| TEXAS INSTRUMENTS INCORPORATED
| Standard Linear and Logic Group
| IBIS Model of TS5A23157
| Dual 10 Ohm SPDT Analog Switch
| This file contains package information for the following:
|  VSSOP 10-pin (DGS) package as [Component] TS5A23157_DGS
| This device can be powered at the following Vccs:
|  5 volt Vcc
|  3.3 volt Vcc
|  2.5 volt Vcc
|  1.8 volt Vcc
| This file provides unique models under the [Model Selector] for each Vcc.
| For operation at a specific Vcc, select the appropriate model after each
| [Model Selector] keyword.
[IBIS Ver]   3.2
[Comment char]  |_char
[File Name]   ts5a23157.ibs
[File Rev]   1.1 | x_die
[Date]   September 27, 2005
[Source]   Data created from TI-SPICE simulations at TI-SLL.
[Notes]   The following is an IBIS list for the TS5A23157.
   Please contact sllibis@ti.com with questions and
   comments concerning SLL IBIS models.
   - FILE REV HISTORY
   - 1.1 Release IBIS file on 10/06/05
   - Power clamp data deleted in the IN models as there
   is no power-clamp diode.
   - Non-monotonic data due to FET characteristics.
   - NCH & PCH MOSFETS, so [Series Mosfet] model can have rising
   or falling currents
[Disclaimer] Property of Texas Instruments Incorporated.  Unauthorized
   reproduction and/or distribution is strictly prohibited.
   This product is protected under copyright law.
   Created  2005, (C) Copyright  2005, Texas Instruments
   Incorporated, All Rights Reserved
   UNLESS THERE IS A SIGNED, WRITTEN AGREEMENT TO THE
   CONTRARY, TEXAS INSTRUMENTS (TI) IS PROVIDING THE IBIS
   MODELS  AND WITHOUT ANY WARRANTY, EXPRESSED OR
   IMPLIED.  TI assumes no liability for:
   1) the accuracy of the IBIS models provided to your
   company;
   2) the proper functioning of these IBIS Models in your
   design or for any resulting applications; or
   3) infringement of patents, copyrights or intellectual
   property rights resulting from your use of these IBIS
   models.
   TI provides IBIS Models as a service to our customers.
   You and your company shall not distribute, sell or give
   these models to anyone else without prior written
   permission from TI.
   TI reserves the right to make changes to our products or
   to discontinue any semiconductor product or service
   without notice, and advises our customers to obtain the
   latest version of relevant information to verify, before
   placing orders, that the information being relied on is
   current.
   Please be aware that your receipt and use of the IBIS
   information provided shall serve as acceptance of these
   terms and conditions.  If you do not accept these terms,
   you should return or destroy the IBIS models and any
   other accompanying information immediately.
| Component TS5A23157_DGS 10-pin VSSOP
[Component]   TS5A23157_DGS
[Manufacturer]   Texas Instruments, Inc.
[Package]
|   typ   min   max
R_pkg   4.300e-02   4.100e-02   4.700e-02
L_pkg   2.235e-09   2.157e-09   2.339e-09
C_pkg   3.350e-13   3.080e-13   3.550e-13
[Pin]   signal_name   model_name   R_pin   L_pin   C_pin
1   IN1   TS5A23157_IN   4.700e-02   2.339e-09   3.100e-13
2   NO1   TS5A23157_NX   4.300e-02   2.213e-09   3.550e-13
3   GND   GND   4.100e-02   2.157e-09   3.540e-13
4   NO2   TS5A23157_NX   4.300e-02   2.213e-09   3.550e-13
5   IN2   TS5A23157_IN   4.700e-02   2.339e-09   3.100e-13
6   COM2   TS5A23157_COM   4.500e-02   2.284e-09   3.080e-13
7   NC2   TS5A23157_NX   4.100e-02   2.176e-09   3.500e-13
8   VCC   POWER   4.100e-02   2.172e-09   3.500e-13
9   NC1   TS5A23157_NX   4.100e-02   2.176e-09   3.510e-13
10   COM1   TS5A23157_COM   4.500e-02   2.284e-09   3.080e-13
[Series Switch Groups]
| Function Group States
On  1 /   | NC1->COM1 IN1 LOW
On  2 /   | NO1->COM1 IN1 HIGH
On  3 /   | NC2->COM2 IN2 LOW
On  4 /   | NO2->COM2 IN2 HIGH
On  5 /   | COM1->NC1 IN1 LOW
On  6 /   | COM1->NO1 IN1 HIGH
On  7 /   | COM2->NC2 IN2 LOW
On  8 /   | COM2->NO2 IN2 HIGH
Off 1 /   | IN1 HIGH
Off 2 /   | IN1 LOW
Off 3 /   | IN2 HIGH
Off 4 /   | IN2 LOW
Off 5 /   | IN1 HIGH
Off 6 /   | IN1 LOW
Off 7 /   | IN2 HIGH
Off 8 /   | IN2 LOW
[Series Pin Mapping]   pin_2   model_name   function_table_group
9   10   TS5A23157_NX_50_S   1
| 9   10   TS5A23157_NX_33_S   1
| 9   10   TS5A23157_NX_25_S   1
| 9   10   TS5A23157_NX_18_S   1
2   10   TS5A23157_NX_50_S   2
| 2   10   TS5A23157_NX_33_S   2
| 2   10   TS5A23157_NX_25_S   2
| 2   10   TS5A23157_NX_18_S   2
7   6   TS5A23157_NX_50_S   3
| 7   6   TS5A23157_NX_33_S   3
| 7   6   TS5A23157_NX_25_S   3
| 7   6   TS5A23157_NX_18_S   3
4   6   TS5A23157_NX_50_S   4
| 4   6   TS5A23157_NX_33_S   4
| 4   6   TS5A23157_NX_25_S   4
| 4   6   TS5A23157_NX_18_S   4
10   9   TS5A23157_COM_50_S   5
| 10   9   TS5A23157_COM_33_S   5
| 10   9   TS5A23157_COM_25_S   5
| 10   9   TS5A23157_COM_18_S   5
10   2   TS5A23157_COM_50_S   6
| 10   2   TS5A23157_COM_33_S   6
| 10   2   TS5A23157_COM_25_S   6
| 10   2   TS5A23157_COM_18_S   6
6   7   TS5A23157_COM_50_S   7
| 6   7   TS5A23157_COM_33_S   7
| 6   7   TS5A23157_COM_25_S   7
| 6   7   TS5A23157_COM_18_S   7
6   4   TS5A23157_COM_50_S   8
| 6   4   TS5A23157_COM_33_S   8
| 6   4   TS5A23157_COM_25_S   8
| 6   4   TS5A23157_COM_18_S   8
| Model TS5A23157_IN
[Model Selector]   TS5A23157_IN
TS5A23157_IN_50   5 volt Vcc
TS5A23157_IN_33   3.3 volt Vcc
TS5A23157_IN_25   2.5 volt Vcc
TS5A23157_IN_18   1.8 volt Vcc
| Model TS5A23157_COM
[Model Selector]   TS5A23157_COM
TS5A23157_COM_50   5 volt Vcc
TS5A23157_COM_33   3.3 volt Vcc
TS5A23157_COM_25   2.5 volt Vcc
TS5A23157_COM_18   1.8 volt Vcc
| Model TS5A23157_COM_S
[Model Selector]   TS5A23157_COM_S
TS5A23157_COM_50_S   5 volt Vcc
TS5A23157_COM_33_S   3.3 volt Vcc
TS5A23157_COM_25_S   2.5 volt Vcc
TS5A23157_COM_18_S   1.8 volt Vcc
| Model TS5A23157_NX
[Model Selector]   TS5A23157_NX
TS5A23157_NX_50   5 volt Vcc
TS5A23157_NX_33   3.3 volt Vcc
TS5A23157_NX_25   2.5 volt Vcc
TS5A23157_NX_18   1.8 volt Vcc
| Model TS5A23157_NX_S
[Model Selector]   TS5A23157_NX_S
TS5A23157_NX_50_S   5 volt Vcc
TS5A23157_NX_33_S   3.3 volt Vcc
TS5A23157_NX_25_S   2.5 volt Vcc
TS5A23157_NX_18_S   1.8 volt Vcc
[Model]   TS5A23157_COM_50_S
Model_type  Series_switch
| variable   typ   min   max
C_comp   0   0   0
[Temperature Range]   40   100   -40
| Ambient temperature   25   85   -40
[Voltage range]   5   4.5   5.5
[On]
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[Off]
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[Model]   TS5A23157_COM_33_S
Model_type  Series_switch
| variable   typ   min   max
C_comp   0   0   0
[Temperature Range]   40   100   -40
| Ambient temperature   25   85   -40
[Voltage range]   3.3   3   3.6
[On]
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[Off]
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[Model]   TS5A23157_COM_25_S
Model_type  Series_switch
| variable   typ   min   max
C_comp   0   0   0
[Temperature Range]   40   100   -40
| Ambient temperature   25   85   -40
[Voltage range]   2.5   2.3   2.7
[On]
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[Off]
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[Model]   TS5A23157_COM_18_S
Model_type  Series_switch
| variable   typ   min   max
C_comp   0   0   0
[Temperature Range]   40   100   -40
| Ambient temperature   25   85   -40
[Voltage range]   1.8   1.65   1.95
[On]
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[Off]
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[Model]   TS5A23157_NX_50_S
Model_type  Series_switch
| variable   typ   min   max
C_comp   0   0   0
[Temperature Range]   40   100   -40
| Ambient temperature   25   85   -40
[Voltage range]   5   4.5   5.5
[On]
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[Off]
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[Model]   TS5A23157_NX_33_S
Model_type  Series_switch
| variable   typ   min   max
C_comp   0   0   0
[Temperature Range]   40   100   -40
| Ambient temperature   25   85   -40
[Voltage range]   3.3   3   3.6
[On]
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[Off]
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[Model]   TS5A23157_NX_25_S
Model_type  Series_switch
| variable   typ   min   max
C_comp   0   0   0
[Temperature Range]   40   100   -40
| Ambient temperature   25   85   -40
[Voltage range]   2.5   2.3   2.7
[On]
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[Off]
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[Model]   TS5A23157_NX_18_S
Model_type  Series_switch
| variable   typ   min   max
C_comp   0   0   0
[Temperature Range]   40   100   -40
| Ambient temperature   25   85   -40
[Voltage range]   1.8   1.65   1.95
[On]
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[Off]
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| Models and submodels in the file (20): TS5A23157_IN_50 (Input), TS5A23157_IN_33 (Input), TS5A23157_IN_25 (Input), TS5A23157_IN_18 (Input), TS5A23157_COM_50_S (Series_switch), TS5A23157_COM_50 (Terminator), TS5A23157_COM_33_S (Series_switch), TS5A23157_COM_33 (Terminator), TS5A23157_COM_25_S (Series_switch), TS5A23157_COM_25 (Terminator), TS5A23157_COM_18_S (Series_switch), TS5A23157_COM_18 (Terminator), TS5A23157_NX_50_S (Series_switch), TS5A23157_NX_50 (Terminator), TS5A23157_NX_33_S (Series_switch), TS5A23157_NX_33 (Terminator), TS5A23157_NX_25_S (Series_switch), TS5A23157_NX_25 (Terminator), TS5A23157_NX_18_S (Series_switch), TS5A23157_NX_18 (Terminator)
